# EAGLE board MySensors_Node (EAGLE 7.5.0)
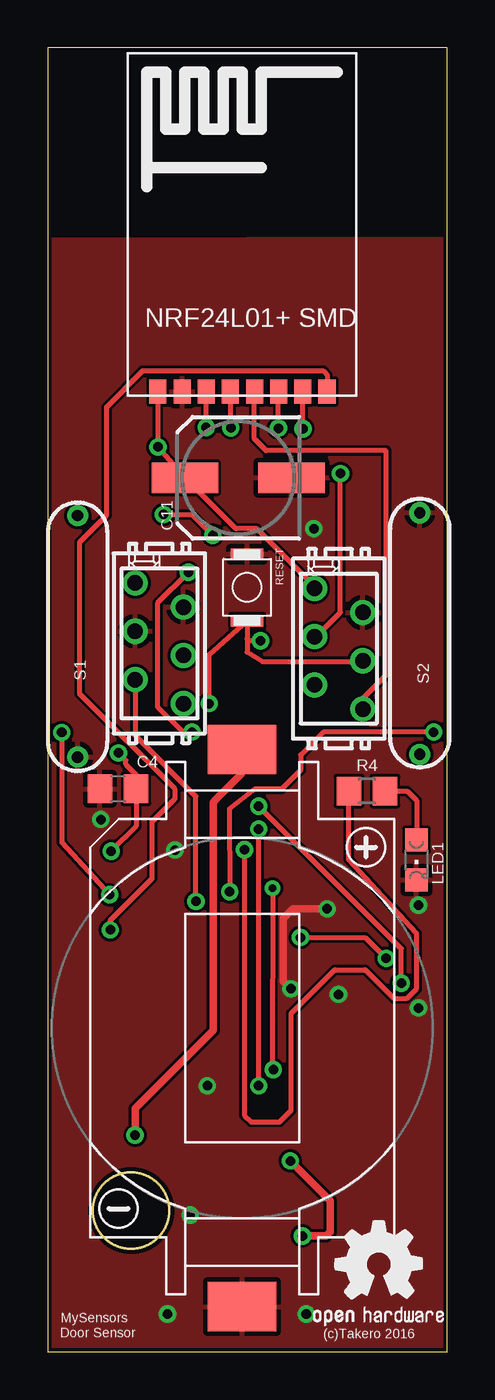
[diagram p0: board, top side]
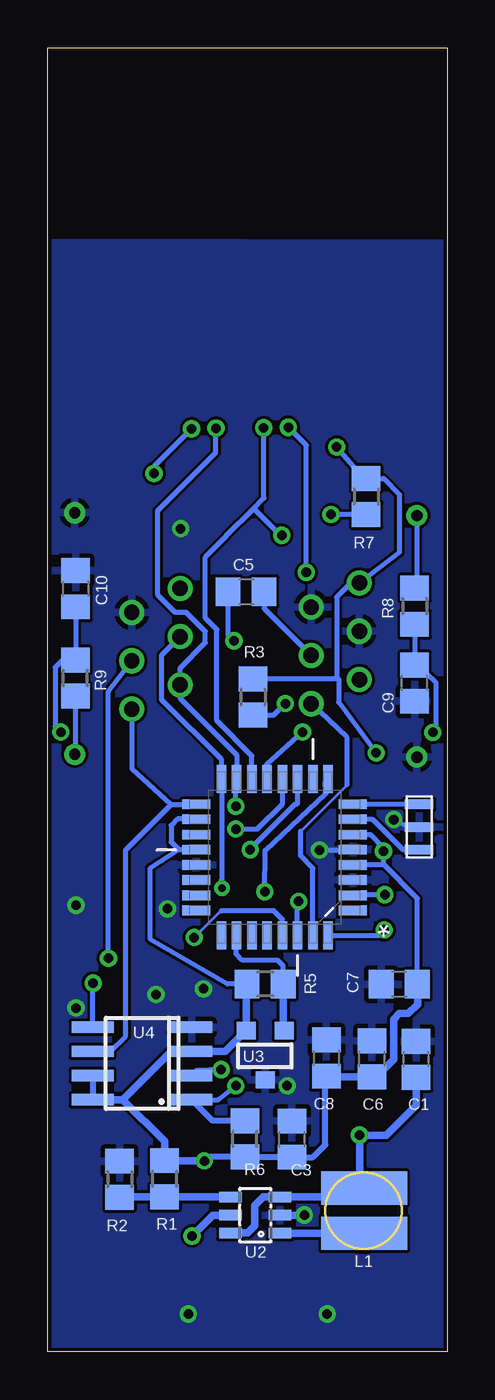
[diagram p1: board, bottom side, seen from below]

Size 21 x 68.6 mm. Coordinates in mm from the lower left corner, seen from the top.
Outline: 0,0 21,0 21,68.6 0,68.6 0,0
Copper layers (1*16): Top 0.035mm / dielectric 1.5mm / Bottom 0.035mm
Design rules "default *": minimum track width 6mil, minimum drill 10mil, track to track 6mil, track to pad 6mil, pad to pad 6mil, via to via 6mil, smd to smd 6mil, copper to edge 8mil, drill to drill 4mil, minimum pad ring 10mil, minimum via ring 8mil, stop-mask expansion 4mil, vias tented up to drill 0mil, thermal gap 10mil

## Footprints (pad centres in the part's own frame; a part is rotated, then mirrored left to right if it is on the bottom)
CH28-2032LF = smd 3.6 x 2.6: NEG 0,-14.65; POS 0,14.65
C0805 = smd 1.3 x 1.5: 1 -0.95,0; 2 0.95,0
SANYO-OSCON_SMD_C6 = smd 3.5 x 1.6: + 2.8,0; - -2.8,0
DLG-0403 = smd 4.5 x 1.75: P$1 0.048,1.189; P$2 0.048,-1.186
CHIPLED_0805 = smd 1.2 x 1.2: A 0,-1.05; C 0,1.05
R0805 = smd 1.3 x 1.5: 1 -0.95,0; 2 0.95,0
B3U-1000P(M) = smd 0.6 x 1.7: 1 -1.75,0; 2 1.75,0
MK6-5 = drill 0.6 pad 1.016: 1 -6.35,0; 2 6.35,0
QFP80P900X900X120-32N = smd 1.473 x 0.508: 1 -4.115,2.794; 2 -4.115,2.007; 3 -4.115,1.194; 4 -4.115,0.406; 5 -4.115,-0.406; 6 -4.115,-1.194; 7 -4.115,-2.007; 8 -4.115,-2.794; 17 4.115,-2.794; 18 4.115,-2.007; 19 4.115,-1.194; 20 4.115,-0.406; 21 4.115,0.406; 22 4.115,1.194; 23 4.115,2.007; 24 4.115,2.794 | smd 0.508 x 1.473: 9 -2.794,-4.115; 10 -2.007,-4.115; 11 -1.194,-4.115; 12 -0.406,-4.115; 13 0.406,-4.115; 14 1.194,-4.115; 15 2.007,-4.115; 16 2.794,-4.115; 25 2.794,4.115; 26 2.007,4.115; 27 1.194,4.115; 28 0.406,4.115; 29 -0.406,4.115; 30 -1.194,4.115; 31 -2.007,4.115; 32 -2.794,4.115
SOT23-6 = smd 0.55 x 1.2: 1 -0.95,-1.3; 2 0,-1.3; 3 0.95,-1.3; 4 0.95,1.3; 5 0,1.3; 6 -0.95,1.3
SOT23-3 = smd 1 x 0.9: 1 -1,-1.3; 2 1,-1.3; 3 0,1.3
SO-08 = smd 0.6 x 2.2: 1 -1.905,-2.6; 2 -0.635,-2.6; 3 0.635,-2.6; 4 1.905,-2.6; 5 1.905,2.6; 6 0.635,2.6; 7 -0.635,2.6; 8 -1.905,2.6
CSTCE = smd 0.5 x 1.5: GND 0,0; IN 1.2,0; OUT -1.2,0
NRF24SMD = smd 0.9 x 1.27: CE -1.27,-6.35; CSN 0,-6.35; GND -2.54,-6.35; IRQ 5.08,-6.35; MISO 3.81,-6.35; MOSI 2.54,-6.35; SCK 1.27,-6.35; VCC -3.81,-6.35
MICROMATCH-6 = drill 0.813: 1 3.175,1.27; 2 1.905,-1.27; 3 0.635,1.27; 4 -0.635,-1.27; 5 -1.905,1.27; 6 -3.175,-1.27

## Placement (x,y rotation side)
BT1  [CH28-2032LF]  10.23,17.04 0 top
C1  [C0805]  1.63,15.39 90 bottom
C3  [C0805]  8.15,11.19 90 bottom
C4  [C0805]  3.7,29.62 180 top
C5  [C0805]  10.56,39.99 0 bottom
C6  [C0805]  3.95,15.42 90 bottom
C7  [C0805]  2.51,19.33 180 bottom
C8  [C0805]  6.35,15.46 270 bottom
C9  [C0805]  1.71,35.18 90 bottom
C10  [C0805]  19.53,40.14 270 bottom
C11  [SANYO-OSCON_SMD_C6]  10.02,45.97 180 top
GOLD_ORB_SM1  OSHWLOGO_GOLD_ORB_SM  [OSHW2]  13.59,0.33 0 top
L1  [DLG-0403]  4.4,7.43 0 bottom
LED1  [CHIPLED_0805]  19.39,25.88 180 top
R1  [R0805]  14.84,9.11 90 bottom
R2  [R0805]  17.21,9.08 270 bottom
R3  [R0805]  10.2,34.44 270 bottom
R4  [R0805]  16.79,29.49 180 top
R5  [R0805]  9.56,19.35 180 bottom
R6  [R0805]  10.62,11.21 90 bottom
R7  [R0805]  4.25,44.98 270 bottom
R8  [R0805]  1.7,39.22 270 bottom
R9  [R0805]  19.54,35.44 90 bottom
RESET  [B3U-1000P(M)]  10.49,40.21 270 top
S1  [MK6-5]  1.58,37.64 90 top
S2  [MK6-5]  19.57,37.78 270 top
U1  [QFP80P900X900X120-32N]  9.06,26.02 180 bottom
U2  [SOT23-6]  10.08,7.2 90 bottom
U3  [SOT23-3]  9.56,15.6 180 bottom
U4  [SO-08]  16.03,15.17 90 bottom
U$1  CSTCE  [CSTCE]  1.46,27.6 270 bottom
U$2  [NRF24SMD]  9.61,56.86 0 top
X1  FTDI  [MICROMATCH-6]  5.87,37.27 90 top
X2  ISP  [MICROMATCH-6]  15.3,36.98 90 top

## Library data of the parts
BT1 = battery-holder
C1 C3-C11 R1-R9 = rcl
GOLD_ORB_SM1 = bfl
L1 = Andi_lib
LED1 = led
RESET = omron
S1 S2 = switch-reed; MF: MEDER; MPN: MK6-5-C; OC_FARNELL: 1079480
U1 = Atmel_By_element14_Batch_1-00; MPN: ATMEGA328P-AU; OC_FARNELL: 1715486; OC_NEWARK: 14R4631; PACKAGE: TQFP-32; SUPPLIER: Atmel
U2 = karlnet-parts
U3 U4 = TD-MySensors
U$1 = murata-cstcc-cstce-cstcr-cstcv-resonators
U$2 = NRF24_SMD
X1 X2 = con-amp-micromatch; MPN: 7-215464-6; OC_FARNELL: 3784630; OC_NEWARK: 19R8125

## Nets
+3V3: C3.1 C4.1 C6.1 C7.1 C8.2 C11.+ R1.2 R3.1 R5.2 R6.1 R7.1 U1.4 U1.6 U1.18 U1.20 U2.5 U3.2 U4.3 U4.7 U4.8 U$2.VCC X1.1 X2.1
A3: R5.1 U1.26 U3.1
B6: U1.7 U$1.IN
B7: U1.8 U$1.OUT
D2: U1.32 U$2.IRQ
D3: U1.1
D4: C9.2 R8.2 U1.2
D5: C10.2 R9.2 U1.9
D6: U1.10
DTR: C5.2 X1.4
FLASH_CSN: R6.2 U1.12 U4.1
FTDI_RX: U1.30 X1.5
FTDI_TX: U1.31 X1.6
GND: BT1.NEG C1.2 C3.2 C4.2 C6.2 C7.2 C8.1 C9.1 C10.1 C11.- LED1.C R2.1 RESET.1 S1.1 S2.1 U1.3 U1.5 U1.21 U2.2 U3.3 U4.4 U$1.GND U$2.GND X1.2 X1.3 X2.2
LED: R4.2 U1.11
MISO: U1.16 U4.2 U$2.MISO X2.3
MOSI: U1.15 U4.5 U$2.MOSI X2.5
N$1: L1.P$2 U2.1
N$2: R1.1 R2.2 U2.4
N$3: BT1.POS C1.1 L1.P$1 U2.3 U2.6
N$4: R8.1 S1.2
N$5: R9.1 S2.2
N$6: LED1.A R4.1
NRF_CE: U1.13 U$2.CE
NRF_CSN: R7.2 U1.14 U$2.CSN
RST: C5.1 R3.2 RESET.2 U1.29 X2.4
SCK: U1.17 U4.6 U$2.SCK X2.6

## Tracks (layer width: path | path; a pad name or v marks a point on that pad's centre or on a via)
+3V3  (via drill 0.5)
  Top 0.254: U$2.VCC v5.8,47.59 C11.+ 9.89,43.3 11,43.3 14.03,40.27 X2.1 | v3.34,26.34 4.65,27.65 C4.1 4.66,29.63 4.66,30.35 4.12,30.9 4.12,31.12 v3.73,31.5
  Top 0.406: v13.4,6.1 14.64,6.1 14.85,6.31 14.85,7.96 v12.76,10.05
  Bottom 0.254: C7.1 1.56,23.86 3.3,25.6 | 3.3,25.6 U1.4 | U1.6 4.01,27.21 3.34,26.54 v3.34,26.34 3.35,26.23 3.35,25.65 3.3,25.6 | R5.2 11.55,19.35 15.6,21.7 15.6,25.44 14.11,26.43 | 14.11,26.43 U1.20 | U1.18 14.18,28.02 14.5,27.7 14.5,26.82 14.11,26.43 | 5.9,35.4 5.7,35.4 5.7,34.18 v3.73,31.5 | 5.9,35.4 R3.1 | 5.9,35.4 5.8,35.5 5.8,39.7 5.06,40.44 X1.1 2.5,42.05 2.5,45.1 3.33,45.93 R7.1 4.34,45.93 v5.8,47.59
  Bottom 0.305: U4.7 U4.8 | v12.76,10.05 12.55,10.26 R6.1 10.61,10.24 C3.1 7.06,10.24 6.4,10.9 6.4,14.46 C8.2
  Bottom 0.406: 17.04,13.27 14.85,11.07 R1.2 14.84,10.05 v12.76,10.05 | 17.04,13.27 U4.8 | 17.04,13.27 14.5,15.81 U4.3 11.66,15.81 U3.2 10.56,19.3 R5.2 | C7.1 1.55,18.28 2.03,17.8 2.5,17.8 2.8,17.5 2.8,15.4 3.73,14.46 C6.1 6.3,14.46 C8.2 | U2.5 12.3,7.2 v13.4,6.1
A3
  Bottom 0.254: R5.1 8.61,20.31 8.9,20.6 10.75,20.6 11.09,20.93 11.09,21.88 U1.26
  Bottom 0.406: R5.1 8.61,16.95 U3.1
B6
  Bottom 0.254: U$1.IN 2.3,26.4 3.9,28 4.92,28 U1.7
B7
  Bottom 0.254: U$1.OUT U1.8
D2  (via drill 0.5)
  Top 0.254: U$2.IRQ 14.71,50.53 14.71,51.37 14.48,51.6 5,51.6 3.1,49.7 3.1,44 1.7,42.6 1.7,34.6 6.7,29.6 6.7,29.1 5.5,27.9 5.5,24.9 3.3,22.7 v3.3,22.2
  Bottom 0.254: U1.32 3.6,21.9 v3.3,22.2
D4  (via drill 0.5)
  Top 0.254: v0.75,32.58 0.75,26.79 v3.27,24.04
  Bottom 0.254: R8.2 C9.2 1.53,36.13 0.6,35.23 0.6,32.73 v0.75,32.58 | v3.27,24.04 4.91,24.04 U1.2
D5  (via drill 0.5)
  Top 0.254: v20.3,32.6 14.5,32.6 13.3,31.4 13.3,30.6 12.3,29.6 10.9,29.6 9.56,28.56 v9.57,24.2
  Bottom 0.254: C10.2 R9.2 20.21,36.39 20.6,36 20.6,32.9 v20.3,32.6 | v9.57,24.2 9.57,26.38 6.37,29.37 6.4,30 U1.9
DTR
  Bottom 0.254: C5.2 9.61,39.1 X1.4
FLASH_CSN  (via drill 0.5)
  Top 0.254: v11.1,14 v11.1,27.5
  Bottom 0.254: U4.1 12.03,13.27 v11.1,14 | v11.1,27.5 9.96,27.5 8.64,28.83 8.64,30.12 U1.12
  Bottom 0.305: R6.2 12.32,12.16 U4.1
FTDI_RX  (via drill 0.5)
  Top 0.254: v7.8,23.7 7.8,29.22 4.6,32.41 X1.5
  Bottom 0.254: U1.30 7.87,23.63 v7.8,23.7
FTDI_TX
  Bottom 0.152: 7.7,27.38 5.25,29.82
  Bottom 0.254: U1.31 7.05,25.45 7.7,26.1 7.7,27.38 | 5.25,29.82 5.26,32.3 X1.6
GND  (via drill 0.5)
  Top 0.406: v14.7,23.3 12.9,23.3 12.4,22.8 12.4,19.5 v12.8,19.1
  Bottom 0.254: U$1.GND 2.1,27.6 v2.8,28 | v6.7,26.4 4.97,26.4 U1.5
  Bottom 0.406: U2.2 v7.5,7.2
  other vias: 6.3,2 13.6,2 8.4,14 19.5,23.5 15.3,18.8 19.5,18.09 14,43.3
  pour Bottom: -0.03,-0.18 21.1,0 21.03,58.36 0.05,58.31
  pour Top: 0.13,-0.15 21.2,0 21.07,58.52 -0.15,58.46
LED  (via drill 0.5)
  Top 0.254: v10.35,26.41 10.35,12.9 10.35,12.45 10.7,12.1 12.2,12.1 12.8,12.7 12.8,17.8 15.1,20.1 16.7,20.1 18.2,18.6 18.9,18.6 19.4,19.1 19.4,22.02 15.82,25.89 15.82,29.47 R4.2
  Bottom 0.254: U1.11 7.87,28.83 7.9,28.8 8,28.8 10.1,26.7 v10.35,26.41
MISO  (via drill 0.4, 0.5)
  Top 0.254: X2.3 14.12,37.62 15.4,38.9 v15.4,46.2 | v13.43,48.55 U$2.MISO | v11.83,24.39 11.81,14.86 v11.87,14.85
  Bottom 0.254: X2.3 15,36.65 15,34.3 11.85,31.15 U1.16 11.85,24.84 v11.83,24.39 | v15.4,46.2 15.4,46.58 v13.43,48.55 | v11.87,14.85 13.17,14.8 U4.2
MOSI  (via drill 0.5)
  Top 0.254: v18.6,19.4 18.6,21.2 v11.1,28.7 | v12.14,48.58 12.14,50.49 U$2.MOSI
  Bottom 0.254: U4.5 18.63,19.37 v18.6,19.4 | v11.1,28.7 11.1,30.1 U1.15 11.06,31.4 14.03,34.37 X2.5 14.03,35.97 12.7,37.3 12.7,37.9 13.7,38.9 14.3,38.9 15.2,39.8 15.2,44.26 12.16,47.29 12.16,48.55 v12.14,48.58
N$1
  Bottom 0.406: U2.1 L1.P$2
N$2
  Bottom 0.406: U2.4 14.83,8.15 R1.1 17.18,8.16 R2.2
N$3  (via drill 0.5)
  Top 0.406: BT1.POS 10.22,31.67 10.22,30.42 8.8,29 8.8,28.99 8.71,28.9 8.71,16.91 4.62,12.82 4.62,11.42 v4.6,11.4
  Bottom 0.406: U2.6 10.47,6.26 10.1,6.63 10.1,7.7 9.65,8.15 U2.3 4.35,8.15 L1.P$1 4.6,8.87 v4.6,11.4 3.2,11.4 1.63,12.97 C1.1
  Bottom 0.813: 4.25,8.72 L1.P$1
N$4
  Bottom 0.254: S1.2 1.58,40.29 R8.1
N$5
  Bottom 0.254: R9.1 19.54,31.47 S2.2
N$6
  Top 0.254: R4.1 18.91,29.5 19.4,29 LED1.A
NRF_CE  (via drill 0.5)
  Top 0.254: v7.6,32.6 7.1,32.6 5.8,33.9 5.8,39.4 v7.4,41 | v8.34,48.63 U$2.CE
  Bottom 0.254: U1.13 9.47,30.93 v7.6,32.6 | v7.4,41 7.4,47.69 v8.34,48.63
NRF_CSN  (via drill 0.5)
  Top 0.254: v9.64,48.6 9.64,50.48 U$2.CSN | v6.1,44.04 7.59,44.04 v8.69,42.95
  Bottom 0.254: U1.14 10.25,31.35 12.1,33.2 12.1,38 12.7,38.6 12.7,41.8 11.6,42.9 11.6,42.92 10.17,44.36 | 10.17,44.36 9.62,44.9 9.62,48.59 v9.64,48.6 | R7.2 6.09,44.03 v6.1,44.04 | v8.69,42.95 8.76,42.95 10.17,44.36
RST  (via drill 0.5)
  Top 0.254: v13.29,21.8 16.7,21.8 v17.8,20.7 | v8.5,34.1 8.5,36.67 RESET.2 10.49,37.5 | 10.49,37.5 10.49,36.81 11.3,36.3 16.12,36.3 X2.4 | v11.2,37.4 10.59,37.4 10.49,37.5
  Bottom 0.152: 11.89,23.19 v13.29,21.8
  Bottom 0.254: U1.29 8.65,22.75 9.1,23.2 11.89,23.19 | v17.8,20.7 17.8,34.72 X2.4 | R3.2 9.11,33.49 v8.5,34.1 | C5.1 11.51,37.71 v11.2,37.4
SCK
  Top 0.254: X2.6 16.57,34.37 17.8,35.6 17.8,47.4 11.49,47.4 10.87,48.02 10.87,50.49 U$2.SCK
  Bottom 0.254: U4.6 17.69,15.81 16.9,16.6 16.9,26.4 14.5,28.8 | 14.5,28.8 13.19,28.8 U1.17 | X2.6 16.57,30.67 14.5,28.8

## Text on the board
tPlace: MySensors | Door Sensor | (c)Takero 2016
